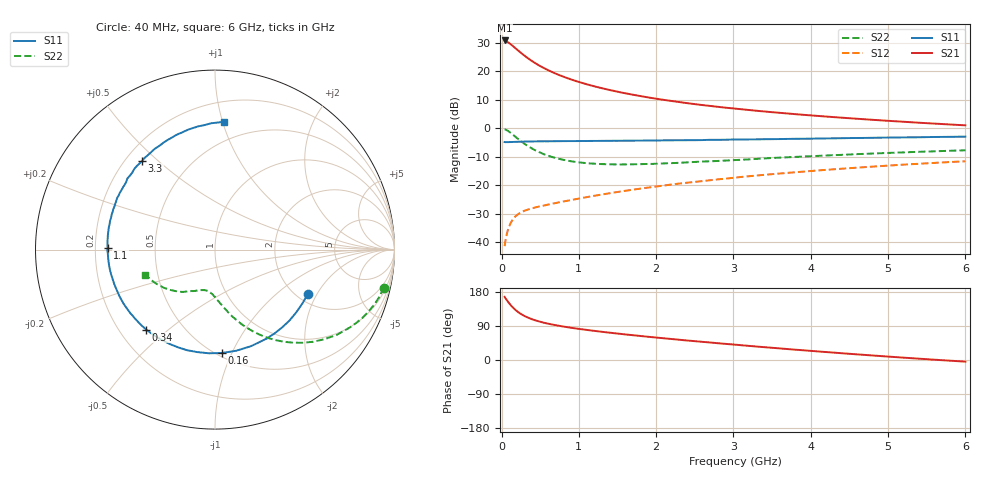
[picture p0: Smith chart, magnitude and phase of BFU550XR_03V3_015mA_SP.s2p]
! Filename:  P:\Prog\Test\Noise\ATS_data\Testdata_Net\03 Spar\BFU550XR_APG2013_45_C05_03p3V_015mA_SP_CM01_D.s2p
! Date/Time: Tue 06/Aug/2013 14:38:14
! BFU550XR_APG2013_45_C05_03p3V_1to35mA_SP_CM01_Bias6_R.s2p
! MDIF S-parameter v. bias file
! BFU550XR_APG2013_45_C05_03p3V_1to35mA_SP_CM01
! Date/time Fri Aug 02 14:41:13 2013
! VAR V_out= 3.3000
! VAR I_out= 14.9950
! VAR V_in= 0.8378
! VAR I_in= 0.1707
! Device data file deembeded for feedlines and parallel
! Original file: \03 Spar\BFU550XR_APG2013_45_C05_03p3V_015mA_SP_CM01_R.s2p
! Feed-files: PR006V01_02082013_Feed1.s2p, PR006V01_02082013_Feed2.s2p
! Parallel-file: PR006V01_02082013_Par.s2p
# MHz S MA R 50
!  Freq-MHz  S11-mag  S11-arg  S21-mag  S21-arg  S12-mag  S12-arg  S22-mag  S22-arg
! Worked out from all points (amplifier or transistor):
!   98 points, 40 MHz to 6 GHz, reference 50 ohm
!   highest |S21| = 30.8 dB at 40 MHz (marker M1)
!   |S21| within 3 dB of that: start of sweep to 191.9 MHz
!   unconditionally stable (mu >= 1): 1.611 GHz to 3.656 GHz
!   at 300 MHz: K = 0.38, MSG = 27.1 dB, |S12| = -28.9 dB
!   at 1.6 GHz: K = 1.00, MSG = 17.1 dB, |S12| = -21.9 dB
!   at 6 GHz: K = 0.88, MSG = 6.3 dB, |S12| = -11.6 dB
!   S11 on the Smith chart (normalised r, x): 40 MHz: 2.29, -1.69; 160 MHz: 0.53, -0.92; 340 MHz: 0.31, -0.42; 1.1 GHz: 0.25, +0.01; 3.3 GHz: 0.27, +0.45; 6 GHz: 0.35, +1.01
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40  0.5741 -25.5  34.63 166.8  0.008592 79.7  0.9643 -12.7
50  0.5718 -31.6  34.29 163.0  0.01052 77.0  0.9534 -15.9
80  0.5727 -49.1  32.37 154.8  0.01608 70.6  0.9054 -24.8
100  0.5735 -59.6  31.01 149.5  0.01926 66.7  0.8671 -30.1
120  0.5743 -69.5  29.66 144.4  0.02208 63.0  0.8284 -35.0
160  0.5772 -86.1  26.68 135.9  0.02669 57.4  0.7488 -43.3
200  0.5794 -99.8  23.99 128.8  0.03018 53.1  0.6744 -50.2
240  0.5821 -110.8  21.62 122.9  0.03283 50.1  0.611 -55.8
280  0.584 -119.8  19.55 118.0  0.03502 48.0  0.5564 -60.5
340  0.5876 -130.7  16.96 112.0  0.03757 46.0  0.4898 -66.1
440  0.5897 -143.9  13.76 104.5  0.04111 44.7  0.4098 -73.0
600  0.592 -157.7  10.49 96.0  0.04594 45.2  0.3313 -80.7
800  0.5961 -169.1  8.033 88.3  0.05218 47.0  0.2807 -87.4
1050  0.5989 -179.3  6.194 80.8  0.06035 49.5  0.2488 -93.5
1100  0.5985 178.9  5.92 79.4  0.06207 49.9  0.2452 -94.6
1500  0.6041 167.0  4.381 69.8  0.0765 52.1  0.233 -101.9
2050  0.6125 154.2  3.221 58.3  0.09724 52.8  0.241 -110.1
3100  0.6379 133.0  2.159 39.0  0.1402 50.1  0.2808 -123.8
3300  0.6398 129.3  2.03 35.5  0.1487 48.9  0.291 -126.1
4100  0.6619 115.5  1.644 22.5  0.1827 44.3  0.3288 -136.3
5200  0.693 97.7  1.302 6.2  0.2308 36.1  0.3785 -150.1
6000  0.7144 85.9  1.127 -4.4  0.2642 29.4  0.4117 -160.2
